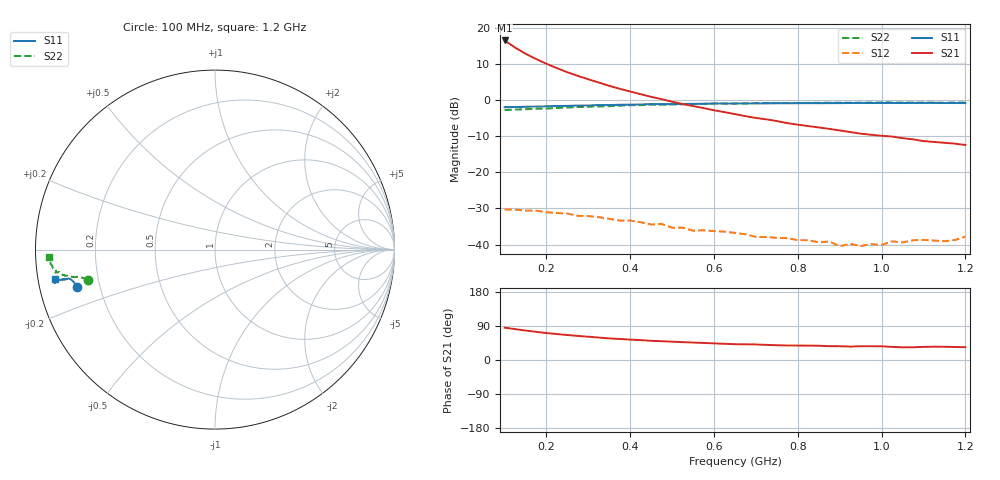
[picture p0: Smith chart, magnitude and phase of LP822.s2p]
!  POLYFET RF DEVICES
!  LP822/LK822  /  L2C 2 Die
!  S PARAMETERS
!  VDS=12.5V, IDQ=400mA
# MHZ S MA R 50
! Freq=Mhz Mag[s11] Ang[s11] Mag[s21] Ang[s21] Mag[s12] Ang[s12] Mag[s22] Ang[s22]
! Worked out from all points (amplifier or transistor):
!   45 points, 100 MHz to 1.2 GHz, reference 50 ohm
!   highest |S21| = 16.5 dB at 100 MHz (marker M1)
!   |S21| within 3 dB of that: start of sweep to 140.1 MHz
!   unconditionally stable (mu >= 1): 533 MHz to 592.3 MHz; 605.4 MHz to end of sweep
!   at 275 MHz: K = 0.40, MSG = 19.4 dB, |S12| = -32.0 dB
!   at 650 MHz: K = 1.35, MAG = 12.9 dB, |S12| = -36.8 dB
!   at 1.2 GHz: K = 3.91, MAG = 3.8 dB, |S12| = -37.8 dB
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100  0.7967 -165.0  6.687 85.3  0.03066 -1.7  0.7295 -166.6
125  0.8021 -166.3  5.33 81.5  0.03041 -5.0  0.7388 -167.3
150  0.8086 -167.2  4.383 77.7  0.02957 -7.4  0.7475 -167.7
175  0.8141 -167.8  3.709 74.4  0.02949 -9.8  0.7584 -168.1
200  0.8204 -168.3  3.178 71.1  0.02807 -11.4  0.7641 -168.4
225  0.8266 -168.6  2.765 68.5  0.0273 -11.5  0.7784 -168.7
250  0.832 -168.9  2.424 65.9  0.02689 -12.2  0.7893 -168.9
300  0.8433 -168.8  1.939 61.4  0.02477 -15.1  0.81 -169.2
350  0.8529 -169.0  1.572 57.0  0.02271 -17.8  0.8242 -169.5
375  0.8624 -168.7  1.431 55.5  0.02149 -15.6  0.8365 -170.0
425  0.8715 -168.9  1.205 52.4  0.02039 -15.4  0.8506 -170.4
475  0.8784 -168.9  1.03 49.5  0.01927 -14.2  0.8641 -170.8
550  0.888 -169.1  0.8268 46.1  0.01558 -13.5  0.8778 -171.9
650  0.8957 -168.9  0.6394 41.7  0.01451 -8.6  0.895 -172.6
850  0.9047 -168.7  0.4181 37.6  0.01075 6.7  0.9168 -174.8
875  0.9072 -168.9  0.3994 36.5  0.01104 14.3  0.9189 -174.9
900  0.9076 -169.1  0.3801 36.4  0.00951 19.8  0.9192 -175.2
925  0.9105 -168.9  0.3612 35.4  0.01021 24.2  0.9188 -175.5
950  0.9139 -168.4  0.3429 36.4  0.00957 32.0  0.9171 -175.8
1025  0.9107 -168.6  0.3128 34.6  0.01108 38.9  0.9277 -176.4
1150  0.9103 -168.7  0.2565 34.9  0.01113 48.8  0.9165 -177.3
1200  0.9085 -169.5  0.2389 33.7  0.01287 56.6  0.9252 -177.6
